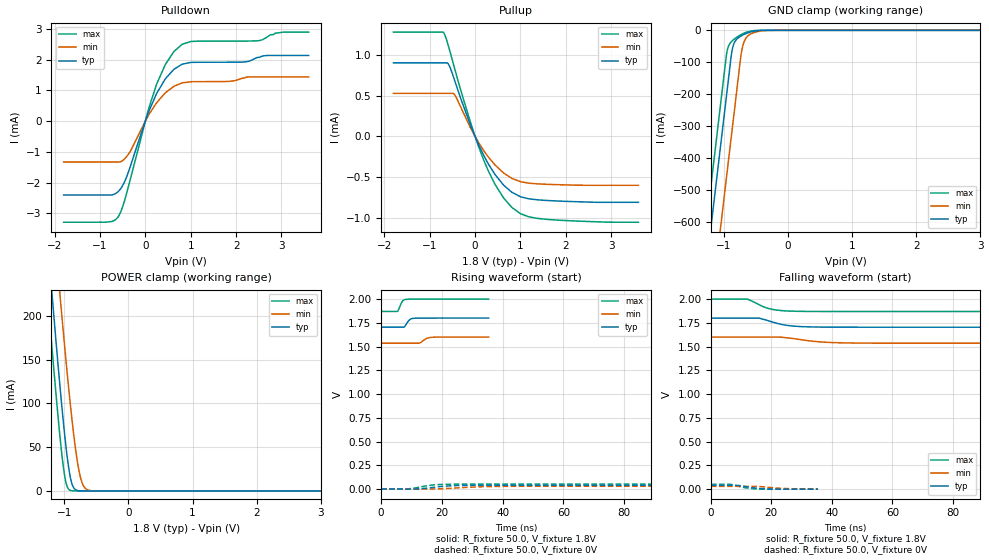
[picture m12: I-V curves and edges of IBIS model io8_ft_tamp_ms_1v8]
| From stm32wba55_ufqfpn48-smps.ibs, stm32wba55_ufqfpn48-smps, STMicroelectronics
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[Model]   io8_ft_tamp_ms_1v8
Model_type I/O
Polarity   Non-Inverting
Enable   Active-Low
| CAP_THRESHOLD on pad IOFT is "UDTCAPC" :
| Rising=30.0% of vddiom   Falling=70.0% of vddiom
| C_comp min and max val. don't necessarily correlate with the min and max pvt
| but are the smallest and greatest pad capacitance found.
| var   typ   min   max
C_comp   6.29605pF  5.93294pF  7.05009pF
|C_comp_pullup   4.08812pF  3.87351pF  4.47686pF
|C_comp_pulldown   2.20793pF  2.05942pF  2.57323pF
Vinl = 800.0mV
Vinh = 1.0V
Vmeas = 900.0mV   | Reference voltage for timing measurements
Cref  = 50.0pF   | Timing specification test load capacitance value
Rref  = 1.0MOhm   | Timing specification test load resistance value
Vref  = 990.0mV   | Timing specification test load voltage
[Model Spec]
| TIME_THRESHOLD on pin ZIV33SW is "CMOS" :
| Rising=50.0% of VDDV33SW   Falling=50.0% of VDDV33SW
Vinl 697.50000mV 636.50000mV 765.50000mV
Vinh 1.08850V 942.50000mV 1.21750V
| variable   typ   min   max
[Temperature Range] 25.0 140.0 -40.0
| variable   typ   min   max
[Voltage Range] 1.8V 1.6V 2.0V
| variable   typ   min   max
[POWER Clamp Reference] 1.8V 1.6V 2.0V
| variable   typ   min   max
[GND Clamp Reference] 0V 0V 0V
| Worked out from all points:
|   slope of the pulldown table from 0 to 0.27 V, typ, clamps not added: 283 ohm
|   slope of the pullup table from 0 to 0.27 V, typ, clamps not added: 855 ohm
|   GND clamp passes 1 mA (typ) near -0.47 V on its own axis
|   POWER clamp passes 1 mA (typ) near -0.81 V on its own axis
|   rising waveform, R_fixture 50.0, V_fixture 1.8V: 20-80 % time 1.33ns typ, 1.85ns min, 1.13ns max; typ from 1.7 V to 1.8 V
|   falling waveform, R_fixture 50.0, V_fixture 1.8V: 20-80 % time 7.15ns typ, 9.98ns min, 5.92ns max; typ from 1.8 V to 1.7 V
[POWER Clamp]
-1.8V     792.8mA    876.2mA    731mA
-1.26V    287mA      389.3mA    225.1mA
-1.19V    224.6mA    328.4mA    163.1mA
-1.06V    114.5mA    218.6mA    57.35mA
-1.02V    83.5mA     186.1mA    30.99mA
-980mV    55.21mA    154.6mA    11.87mA
-910mV    17.39mA    102.5mA    764.6uA
-850mV    3.285mA    62.83mA    47.95uA
-760mV    138.8uA    19.43mA    717.2nA
-700mV    15.66uA    5.838mA    43.61nA
-620mV    848.9nA    820.4uA    1.186nA
3.6V      0A         0A         0A
[GND Clamp]
-1.8V     -1.639A    -1.894A    -1.509A
-1.43V    -1.01A     -1.265A    -879.6mA
-1.24V    -686.9mA   -942.2mA   -556.6mA
-1.05V    -363.9mA   -619.2mA   -233.6mA
-950mV    -193.9mA   -449.2mA   -67.62mA
-870mV    -63.28mA   -313.2mA   -33.62mA
-820mV    -33.62mA   -228.2mA   -25.22mA
-730mV    -17.72mA   -77.21mA   -13.43mA
-690mV    -13.46mA   -40.36mA   -9.392mA
-630mV    -8.329mA   -18.75mA   -4.815mA
-370mV    -86.03uA   -1.078mA   -3.689uA
3.6V      2.71nA     3.15uA     1.142nA
| variable   typ   min   max
[Pullup Reference] 1.8V 1.6V 2.0V
| variable   typ   min   max
[Pulldown Reference] 0V 0V 0V
[Pullup]
-1.8V     905.2uA    529.7uA    1.283mA
-690mV    905.2uA    529.7uA    1.273mA
-590mV    891uA      529.7uA    1.118mA
-450mV    688.6uA    513uA      834.2uA
-120mV    167uA      126.5uA    207uA
160mV     -198uA     -148.3uA   -248.1uA
440mV     -469.3uA   -352.1uA   -590.3uA
630mV     -600.6uA   -451uA     -758.9uA
810mV     -687.5uA   -516.3uA   -873.7uA
1V        -742.6uA   -557.2uA   -950.7uA
1.37V     -780.2uA   -583.9uA   -1.008mA
3.6V      -810.9uA   -601.5uA   -1.056mA
[Pulldown]
-1.8V     -2.401mA   -1.328mA   -3.284mA
-870mV    -2.401mA   -1.328mA   -3.284mA
-600mV    -2.291mA   -1.328mA   -3.111mA
-490mV    -2.066mA   -1.268mA   -2.736mA
-350mV    -1.554mA   -1.026mA   -1.996mA
60mV      249uA      165uA      332.9uA
250mV     902.8uA    602.2uA    1.206mA
440mV     1.374mA    920.6uA    1.837mA
810mV     1.85mA     1.242mA    2.495mA
2.46V     2.065mA    1.435mA    2.609mA
2.87V     2.134mA    1.435mA    2.859mA
3.6V      2.134mA    1.435mA    2.893mA
[Ramp]
dV/dt_r 23.80839mV/7.24659ns 17.67402mV/11.15561ns 31.02286mV/5.51241ns
dV/dt_f 57.44931mV/7.10888ns 38.53683mV/9.87139ns 78.08536mV/5.71799ns
R_load = 50.0
| Removed startup time: 0s 0s 0s  .
| Removed end time: 35.4ns.
[Rising Waveform]
R_fixture   = 50.0
V_fixture   = 1.8V
V_fixture_min = 1.6V
V_fixture_max = 2.0V
0s        1.704V     1.536V     1.87V
5.35ns    1.704V     1.536V     1.87V
7ns       1.704V     1.536V     1.976V
8.1ns     1.727V     1.536V     1.997V
9.45ns    1.784V     1.536V     1.999V
10.85ns   1.798V     1.536V     2V
13ns      1.799V     1.541V     2V
14.7ns    1.8V       1.581V     2V
16.65ns   1.8V       1.597V     2V
35.4ns    1.8V       1.6V       2V
| Removed startup time: 0s 0s 0s  .
| Removed end time: 198.4ns.
[Falling Waveform]
R_fixture   = 50.0
V_fixture   = 1.8V
V_fixture_min = 1.6V
V_fixture_max = 2.0V
0s        1.8V       1.6V       2V
12.15ns   1.8V       1.6V       2V
16.2ns    1.798V     1.6V       1.937V
17.85ns   1.783V     1.6V       1.914V
20.2ns    1.76V      1.6V       1.893V
24.45ns   1.727V     1.595V     1.876V
29.1ns    1.712V     1.576V     1.871V
37.65ns   1.705V     1.546V     1.87V
48.6ns    1.704V     1.537V     1.87V
198.4ns   1.704V     1.536V     1.87V
| Removed startup time: 0s 0s 0s  .
| Removed end time: 198.35ns.
[Rising Waveform]
R_fixture   = 50.0
V_fixture   = 0V
V_fixture_min = 0V
V_fixture_max = 0V
0s        26.35nV    4.279uV    25.49nV
8.1ns     -1.237mV   4.274uV    -967.3uV
12.15ns   1.792mV    27.92uV    16.03mV
14.9ns    8.66mV     -906.2uV   33.45mV
17.35ns   18.02mV    555.6uV    43.3mV
21.25ns   30.33mV    5.055mV    49.49mV
24.45ns   35.48mV    10.43mV    51.14mV
33.25ns   39.3mV     23.87mV    51.71mV
44.35ns   39.67mV    28.73mV    51.72mV
198.3ns   39.68mV    29.46mV    51.7mV
| Removed startup time: 0s 0s 0s  .
| Removed end time: 35.4ns.
[Falling Waveform]
R_fixture   = 50.0
V_fixture   = 0V
V_fixture_min = 0V
V_fixture_max = 0V
0s        39.68mV    29.47mV    51.71mV
6.35ns    39.68mV    29.47mV    51.4mV
9.1ns     39.02mV    29.47mV    30.69mV
11.75ns   25.43mV    29.47mV    12.2mV
13.4ns    17.21mV    29.47mV    5.906mV
15.35ns   9.278mV    29.49mV    1.495mV
19.55ns   1.517mV    17.65mV    198.4uV
23.15ns   249.1uV    8.792mV    44.84uV
29.65ns   30.37uV    1.438mV    1.624uV
35.4ns    3.834uV    356.9uV    -524nV
